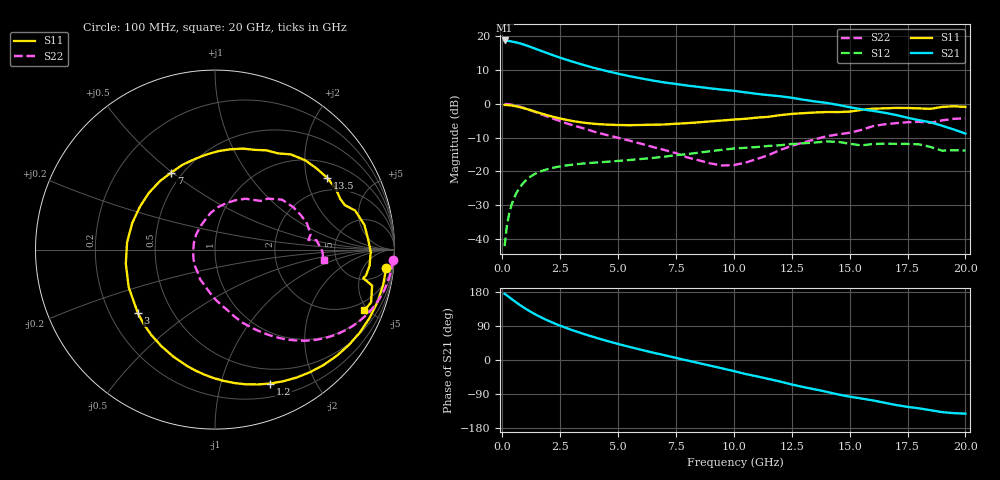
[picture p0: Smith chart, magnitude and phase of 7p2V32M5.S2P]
! Infineon Technologies  Discrete & RF Semiconductors
! bfp620
! VCE =  2.3 V,  IC =  2.5 mA
! Common Emitter S-Parameters:  Sep 2002
# GHz  S  MA  R  50
!  f  S11  S21  S12  S22
! GHz  MAG  ANG  MAG  ANG  MAG  ANG  MAG  ANG
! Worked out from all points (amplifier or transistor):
!   59 points, 100 MHz to 20 GHz, reference 50 ohm
!   highest |S21| = 18.7 dB at 100 MHz (marker M1)
!   |S21| within 3 dB of that: start of sweep to 1.646 GHz
!   unconditionally stable (mu >= 1): 5.489 GHz to 13.4 GHz; 14.2 GHz to 15.58 GHz; 17.54 GHz to end of sweep
!   at 1 GHz: K = 0.19, MSG = 20.1 dB, |S12| = -22.8 dB
!   at 5.5 GHz: K = 1.00, MAG = 12.2 dB, |S12| = -16.7 dB
!   at 20 GHz: K = 1.30, MAG = -0.8 dB, |S12| = -13.9 dB
!   S11 on the Smith chart (normalised r, x): 100 MHz: 6, -16; 1.2 GHz: 0.34, -1.44; 3 GHz: 0.32, -0.33; 7 GHz: 0.44, +0.49; 13.5 GHz: 1.50, +2.66; 20 GHz: 1.35, -4.75
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0.1  0.9597 -6.1  8.643 174.7  0.0078 79.1  0.9928 -3.5
0.2  0.9572 -12.0  8.549 170.3  0.0159 80.5  0.9883 -7.0
0.4  0.9418 -23.9  8.342 161.0  0.0319 75.8  0.9686 -13.8
0.7  0.9001 -41.1  7.922 147.7  0.0539 66.3  0.9185 -23.4
0.9  0.8647 -52.1  7.563 139.5  0.0667 60.1  0.8761 -29.2
1.2  0.8072 -67.6  6.969 128.2  0.0825 51.7  0.8066 -36.8
1.6  0.7324 -86.4  6.202 114.9  0.098 42.4  0.7157 -45.2
2  0.6671 -103.4  5.523 103.3  0.1088 35.0  0.6361 -51.8
2.4  0.6154 -119.0  4.934 92.9  0.1167 29.0  0.5682 -57.3
3  0.5571 -140.4  4.226 79.2  0.125 21.9  0.4857 -64.4
3.5  0.5249 -156.3  3.76 69.0  0.1306 17.2  0.4333 -69.6
4  0.5031 -171.0  3.368 59.6  0.1344 13.1  0.3829 -74.3
5  0.4842 162.2  2.783 42.3  0.1426 7.4  0.314 -82.9
6  0.4853 139.4  2.372 26.9  0.1523 2.6  0.2557 -93.9
7  0.4934 119.7  2.067 12.7  0.1646 -1.8  0.2069 -106.4
8.5  0.5312 95.5  1.772 -8.3  0.1893 -10.2  0.1452 -139.6
10.5  0.5992 68.0  1.474 -36.9  0.2228 -26.2  0.1345 141.4
12  0.678 51.5  1.291 -56.9  0.2431 -37.4  0.2064 96.6
13.5  0.7421 32.6  1.081 -77.4  0.2668 -51.5  0.2972 67.6
15  0.7648 18.9  0.889 -96.7  0.2554 -70.9  0.372 46.8
17  0.8677 -0.9  0.682 -118.7  0.2551 -83.0  0.516 21.7
20  0.8988 -22.1  0.362 -141.5  0.2023 -102.6  0.6082 -5.6
